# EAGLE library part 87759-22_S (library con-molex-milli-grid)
HEADER
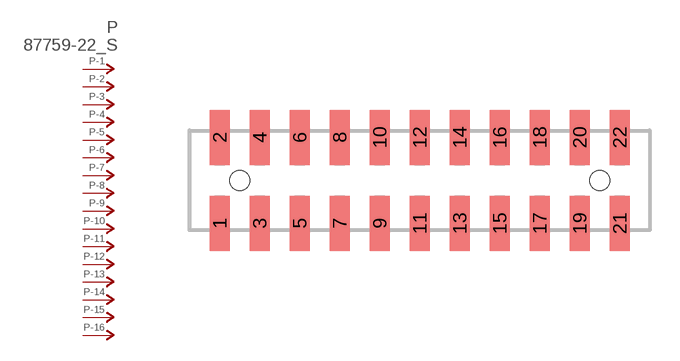
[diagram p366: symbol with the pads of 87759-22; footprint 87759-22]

Designator prefix P; gates -1=P-NV -2=P-N -3=P-N -4=P-N -5=P-N -6=P-N -7=P-N -8=P-N -9=P-N -10=P-N -11=P-N -12=P-N -13=P-N -14=P-N -15=P-N -16=P-N -17=P-N -18=P-N -19=P-N -20=P-N -21=P-N -22=P-N

## 87759-22_S  [87759-22]
1  -1:P  pas
2  -2:P  pas
3  -3:P  pas
4  -4:P  pas
5  -5:P  pas
6  -6:P  pas
7  -7:P  pas
8  -8:P  pas
9  -9:P  pas
10  -10:P  pas
11  -11:P  pas
12  -12:P  pas
13  -13:P  pas
14  -14:P  pas
15  -15:P  pas
16  -16:P  pas
17  -17:P  pas
18  -18:P  pas
19  -19:P  pas
20  -20:P  pas
21  -21:P  pas
22  -22:P  pas

## Footprint 87759-22 (pad centres in mm)
HEADER SMD Dual Row, Vertical
smd 1 x 2.75: 1 -10,-2.15; 2 -10,2.15; 3 -8,-2.15; 4 -8,2.15; 5 -6,-2.15; 6 -6,2.15; 7 -4,-2.15; 8 -4,2.15; 9 -2,-2.15; 10 -2,2.15; 11 0,-2.15; 12 0,2.15; 13 2,-2.15; 14 2,2.15; 15 4,-2.15; 16 4,2.15; 17 6,-2.15; 18 6,2.15; 19 8,-2.15; 20 8,2.15; 21 10,-2.15; 22 10,2.15
hole 1 at -9,0
hole 1 at 9,0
